FUNCTION_BLOCK FB_EtherCATDiag
VAR_INPUT
	sIPCNetID					: T_AmsNetId; 	// AmsNetId of the IPC 
	sMasterNetID				: T_AmsNetId; 	// AmsNetId of the EtherCAT master device 
	nMasterDevID				: UINT;			// Device ID of EtherCAT master
	nSlaveCount 				: UINT;			// current slave count
	nSlaveCountCfg 				: UINT;			// configured slave count
	nMasterDevState				: WORD;			// device state of EtherCAT Master
	bAllFrameWcStatesOK			: BOOL;			// all FrameWcState OK?
	tTimeout					: TIME := T#5S; // ads timeout
END_VAR
VAR_OUTPUT
	bEtherCATOK					: BOOL;			// no problem on EtherCAT
	bFrameWcStateError			: BOOL;			// error in at least one frame
	bSlaveCountError			: BOOL;			// EtherCAT slave count mismatch (# of cfg slaves <> # of found slaves)
	bMasterDevStateError		: BOOL;			// error in master device state
	stMasterDevState			: ST_EcMasterDevState; // splitted master device state
	bBusy						: BOOL;			// FB busy
	bError						: BOOL;			// FB with error
	iErrorID					: UDINT;		// FB error ID
END_VAR
VAR_IN_OUT
	arrDiagSlaveInfo 			: ARRAY [0..3] OF ST_SlaveStateInfo;		// read in info from configured slaves
	arrDiagSlaveInfoScanned		: ARRAY [0..3] OF ST_SlaveStateInfoScanned;	// read in info from scanned slaves
END_VAR
VAR
	iState						: INT;
	nMasterDevStatePrev			: WORD;
	bSlaveCountErrorPrev		: BOOL;
	bAllFrameWcStatesOKPrev		: BOOL;
	bDiagReq					: BOOL := TRUE;
	I							: UDINT;

	(* -- Get Slave Addresses *)
	fbGetSlaveAddresses 		: FB_EcGetAllSlaveAddr;
	arrSlaveAddresses 			: ARRAY[0..iSLAVEADDR_ARR_SIZE] OF UINT;
	iNumOfSlavesRead			: UINT;

	(* -- Get Slave States *)
	fbGetAllSlaveStates			: FB_EcGetAllSlaveStates;
	arrSlaveStates 				: ARRAY[0..iSLAVEADDR_ARR_SIZE] OF ST_EcSlaveState;

	(* -- Get Topology Data *)
	iTopologyData				: UDINT;
	fbGetTopologyData			: ADSREAD;
	arrTopologyData				: ARRAY[0..iSLAVEADDR_ARR_SIZE] OF ST_TopologyData;

	(* -- Check Topology *)
	iDiagIndex					: ARRAY [0..3] OF UINT;
	iDiagPort					: ARRAY [0..3] OF UINT;
	iIdx						: DINT;

	(* -- Scan Slaves *)
	fbEcGetScannedSlaves		: FB_EcGetScannedSlaves;
	arrScannedSlaveInfo			: ARRAY [0..iSLAVEADDR_ARR_SIZE] OF ST_EcSlaveScannedData;
	nScannedSlaves				: UINT;

	(* -- Get Slave Identities *)
	fbGetSlaveIdentity			: FB_EcGetSlaveIdentity;
	stIdentity 					: ST_EcSlaveIdentity;

	(* -- Get Slave Names *)
	fbGetSlaveName 				: IOF_GetBoxNameByAddr;
	strName						: STRING;

	arrSlaveInfo 				: ARRAY [0..iSLAVEADDR_ARR_SIZE] OF ST_SlaveStateInfo;
	arrSlaveInfoScanned			: ARRAY [0..iSLAVEADDR_ARR_SIZE] OF ST_SlaveStateInfoScanned;
END_VAR

(* cyclic diag *)
bFrameWcStateError := NOT bAllFrameWcStatesOK;

bSlaveCountError := (nSlaveCount <> nSlaveCountCfg) OR (nSlaveCount = 0);
IF (bSlaveCountError AND NOT bSlaveCountErrorPrev) OR (NOT bSlaveCountError AND bSlaveCountErrorPrev) THEN
	bSlaveCountErrorPrev := bSlaveCountError;
	bDiagReq := TRUE; // slave count error change detected --> diag required
END_IF

IF (bAllFrameWcStatesOK AND NOT bAllFrameWcStatesOKPrev) OR (NOT bAllFrameWcStatesOK AND bAllFrameWcStatesOKPrev) THEN
	bAllFrameWcStatesOKPrev := bAllFrameWcStatesOK;
	bDiagReq := TRUE; // frame error change detected --> diag required
END_IF

IF (nMasterDevState <> nMasterDevStatePrev) THEN
	M_CheckMasterDevState();
	bDiagReq := TRUE; // devstate change detected --> diag required
END_IF

(* acyclic diag *)
CASE iState OF
0: (* IDLE *)
	IF bDiagReq THEN				// diag requested
		bDiagReq := FALSE;

		IF sMasterNetID <> '' AND sMasterNetID <> '0.0.0.0.0.0' THEN
			iState := iState + 1;	// execute diag
			bBusy := TRUE;
		ELSE
			bError := TRUE;
			iErrorID := 7;
		END_IF

		bEtherCATOK := FALSE;
	ELSE
		// check for changes in idle
		IF (bSlaveCountError OR bMasterDevStateError OR NOT bAllFrameWcStatesOK) AND NOT (arrSlaveInfo[iDiagIndex[0]].bDiagData) THEN
			bEtherCATOK := FALSE;
			bDiagReq := TRUE;//new error --> diag requested
		ELSIF (bSlaveCountError AND NOT bSlaveCountErrorPrev) OR (NOT bSlaveCountError AND bSlaveCountErrorPrev) THEN
			bSlaveCountErrorPrev := bSlaveCountError;
			bEtherCATOK := FALSE;
			bDiagReq := TRUE;// slave count error change detected --> diag required
		ELSIF (nMasterDevState <> nMasterDevStatePrev) THEN
			bEtherCATOK := FALSE;
			bDiagReq := TRUE;// devstate change detected --> diag required
		ELSIF (bAllFrameWcStatesOK AND NOT bAllFrameWcStatesOKPrev) OR (NOT bAllFrameWcStatesOK AND bAllFrameWcStatesOKPrev) THEN
			bAllFrameWcStatesOKPrev := bAllFrameWcStatesOK;
			bEtherCATOK := FALSE;
			bDiagReq := TRUE;// frame error change detected --> diag required
		ELSIF (bSlaveCountError OR bMasterDevStateError OR NOT bAllFrameWcStatesOK OR arrSlaveInfo[iDiagIndex[0]].bDiagData) THEN
			bEtherCATOK := FALSE;
		ELSE
			bEtherCATOK := TRUE;
		END_IF
	END_IF

1: (* get adresses *)
	M_GetSlaveAdresses();

2: (* get states *)
	M_GetSlaveStates();

3:	(* get topology data length *)
	M_GetTopoDataLen();

4:	(* get topology data *)
	M_GetTopoData();

5:	(* scan slaves *)
	M_ScanSlaves();

6:	(* get identity *)
	M_GetSlaveIdentity();

7:	(* get name *)
	M_GetSlaveName();

8:	(* get scanned name *)
	M_GetScannedSlaveName();

10:	(* DONE *)
	bBusy := FALSE;
	iState := 0;


END_CASE

ACTION M_GetSlaveAdresses:
fbGetSlaveAddresses(
	sNetId		:= sMasterNetID,
	pAddrBuf	:= ADR(arrSlaveAddresses),
	cbBufLen	:= SIZEOF(arrSlaveAddresses),
	bExecute	:= TRUE,
	tTimeout	:= tTimeout,
	nSlaves		=> iNumOfSlavesRead
);

IF NOT fbGetSlaveAddresses.bBusy THEN
	fbGetSlaveAddresses(bExecute:= FALSE);
	IF NOT fbGetSlaveAddresses.bError THEN
		FOR I := 0 TO MIN(iNumOfSlavesRead, iSLAVEADDR_ARR_SIZE) DO
			arrSlaveInfo[I].nECAddr := arrSlaveAddresses[I];
		END_FOR
	END_IF
	iState := iState + 1;
END_IF
END_ACTION

ACTION M_GetSlaveName:
fbGetSlaveName(
	NETID		:= sIPCNetId,
	DEVICEID	:= nMasterDevID,
	BOXADDR		:= arrSlaveInfo[iDiagIndex[iIdx]].nECAddr,
	START		:= TRUE,
	TMOUT		:= tTimeout,
	BOXNAME		=> strName
);

IF NOT fbGetSlaveName.BUSY THEN
	fbGetSlaveName(START:= FALSE);

	IF NOT fbGetSlaveName.ERR THEN
		IF iDiagPort[iIdx] <> 0 THEN
			arrSlaveInfo[iDiagIndex[iIdx]].sName 	:= strName;
		END_IF
	END_IF

	iState := iState + 1;
END_IF
END_ACTION

ACTION M_GetSlaveIdentity:
fbGetSlaveIdentity(
	sNetId		:= sMasterNetID,
	nSlaveAddr	:= arrSlaveInfo[iDiagIndex[iIdx]].nECAddr,
	bExecute	:= TRUE,
	tTimeout	:= tTimeout,
	identity	=> stIdentity
);

IF NOT fbGetSlaveIdentity.bBusy THEN
	fbGetSlaveIdentity(bExecute:= FALSE);

	IF NOT fbGetSlaveIdentity.bError THEN
		IF iDiagPort[iIdx] <> 0 THEN
			arrSlaveInfo[iDiagIndex[iIdx]].nIndex	:= iDiagIndex[iIdx] + 1;
			arrSlaveInfo[iDiagIndex[iIdx]].sType 	:= F_ConvProductCodeToString(stSlaveIdentity := stIdentity);
		END_IF
	END_IF
	iState := iState + 1;
END_IF
END_ACTION

ACTION M_ScanSlaves:
fbEcGetScannedSlaves(
	bExecute				:= TRUE,
	sNetId					:= sMasterNetID,
	pArrEcScannedSlaveInfo	:= ADR(arrScannedSlaveInfo),
	cbBufLen				:= SIZEOF(arrScannedSlaveInfo),
	tTimeout				:= tTimeout
);

IF NOT fbEcGetScannedSlaves.bBusy THEN
	fbEcGetScannedSlaves(bExecute := FALSE);
	iState := iState + 1;

	IF fbEcGetScannedSlaves.bError THEN
		nScannedSlaves := 0;
	ELSE
		nScannedSlaves := fbEcGetScannedSlaves.nSlaves;
	END_IF
END_IF
END_ACTION

ACTION M_GetScannedSlaveName:
fbGetSlaveName(
	NETID		:= sIPCNetId,
	DEVICEID	:= nMasterDevID,
	BOXADDR		:= arrScannedSlaveInfo[iDiagIndex[iIdx]].nAddr,
	START		:= TRUE,
	TMOUT		:= tTimeout,
	BOXNAME		=> strName
);

IF NOT fbGetSlaveName.BUSY THEN
	fbGetSlaveName(START:= FALSE);

	(* add scanned info *)
	arrSlaveInfoScanned[iDiagIndex[iIdx]].nIndex 	:= iDiagIndex[iIdx] + 1;
	IF arrScannedSlaveInfo[iDiagIndex[iIdx]].nAddr <> 0 THEN
		IF NOT fbGetSlaveName.ERR THEN
			arrSlaveInfoScanned[iDiagIndex[iIdx]].sName := strName;
		END_IF
	ELSE
		arrSlaveInfoScanned[iDiagIndex[iIdx]].sType		:= '';
	END_IF

	IF (iDiagIndex[iIdx] < nScannedSlaves) THEN
		arrSlaveInfoScanned[iDiagIndex[iIdx]].sType		:= F_ConvProductCodeToString(arrScannedSlaveInfo[iDiagIndex[iIdx]].stSlaveIdentity);
	ELSE
		arrSlaveInfoScanned[iDiagIndex[iIdx]].sType		:= '';
	END_IF

	arrSlaveInfoScanned[iDiagIndex[iIdx]].nECAddr	:= arrScannedSlaveInfo[iDiagIndex[iIdx]].nAddr;

	IF arrSlaveInfoScanned[iDiagIndex[iIdx]].sName <> arrSlaveInfo[iDiagIndex[iIdx]].sName THEN
		arrSlaveInfoScanned[iDiagIndex[iIdx]].bDifferentName := TRUE;
	ELSE
		arrSlaveInfoScanned[iDiagIndex[iIdx]].bDifferentName := FALSE;
	END_IF

	IF arrSlaveInfoScanned[iDiagIndex[iIdx]].nECAddr <> arrSlaveInfo[iDiagIndex[iIdx]].nECAddr THEN
		arrSlaveInfoScanned[iDiagIndex[iIdx]].bDifferentAddr := TRUE;
	ELSE
		arrSlaveInfoScanned[iDiagIndex[iIdx]].bDifferentAddr := FALSE;
	END_IF

	IF arrSlaveInfoScanned[iDiagIndex[iIdx]].sType <> arrSlaveInfo[iDiagIndex[iIdx]].sType THEN
		arrSlaveInfoScanned[iDiagIndex[iIdx]].bDifferentType := TRUE;
	ELSE
		arrSlaveInfoScanned[iDiagIndex[iIdx]].bDifferentType := FALSE;
	END_IF

	IF iIdx < 3 THEN
		iIdx := iIdx + 1;
		iState := iState - 2;
	ELSE
		iIdx := 0;
		iState := 10;

		FOR I := 0 TO 3 DO
			IF iDiagPort[I] <> 0 THEN
				arrDiagSlaveInfo[I] := arrSlaveInfo[iDiagIndex[I]];
				arrDiagSlaveInfoScanned[I] := arrSlaveInfoScanned[iDiagIndex[I]];
			ELSE
				MEMSET(ADR(arrDiagSlaveInfo[I]), 0, SIZEOF(arrDiagSlaveInfo[I]));
				MEMSET(ADR(arrDiagSlaveInfoScanned[I]), 0, SIZEOF(arrDiagSlaveInfoScanned[I]));
			END_IF
		END_FOR
	END_IF
END_IF
END_ACTION

ACTION M_CheckMasterDevState:
(* check master errors based on devstate *)
bMasterDevStateError 				:= nMasterDevState <> 0;
stMasterDevState.bLinkError 		:= ((nMasterDevState AND 16#000F) = 1) OR ((nMasterDevState AND 16#000F) = 4);
stMasterDevState.bResetRequired 	:= ((nMasterDevState AND 16#000F) = 2) OR ((nMasterDevState AND 16#FFF0) = 16#10);
stMasterDevState.bMissFrmRedMode 	:= (nMasterDevState AND 16#000F) = 8;
stMasterDevState.bWatchdogTriggerd 	:= (nMasterDevState AND 16#20) = 16#20;
stMasterDevState.bDriverNotFound 	:= (nMasterDevState AND 16#40) = 16#40;
stMasterDevState.bResetActive 		:= (nMasterDevState AND 16#80) = 16#80;
stMasterDevState.bAtLeastOneNotInOp := ((nMasterDevState AND 16#100) = 16#100) OR ((nMasterDevState AND 16#200) = 16#200) OR
										((nMasterDevState AND 16#400) = 16#400) OR ((nMasterDevState AND 16#800) = 16#800);
stMasterDevState.bDcNotInSync 		:= (nMasterDevState AND 16#1000) = 16#1000;
nMasterDevStatePrev 				:= nMasterDevState;
END_ACTION

ACTION M_GetTopoData:
fbGetTopologyData(
	NETID	:= sMasterNetID,
	PORT	:= 16#FFFF,
	IDXGRP	:= 16#22,
	IDXOFFS	:= 0,
	LEN		:= iTopologyData*SIZEOF(arrTopologyData[0]),
	DESTADDR:= ADR(arrTopologyData),
	READ	:= TRUE,
	TMOUT	:= tTimeout,
);

IF NOT fbGetTopologyData.BUSY THEN
	fbGetTopologyData(READ := FALSE);

	IF NOT fbGetTopologyData.ERR THEN
		iDiagPort[0] := arrTopologyData[iDiagIndex[0]].iOwnPhysicalAddr;
		iDiagPort[1] := arrTopologyData[iDiagIndex[0]].stPhysicalAddr.portB;
		iDiagPort[2] := arrTopologyData[iDiagIndex[0]].stPhysicalAddr.portC;
		iDiagPort[3] := arrTopologyData[iDiagIndex[0]].stPhysicalAddr.portD;

		(* clear diag index  *)
		iDiagIndex[1] := 0;
		iDiagIndex[2] := 0;
		iDiagIndex[3] := 0;

		(* find slaves on PortB of first slave with diag *)
		IF iDiagPort[1] <> 0 THEN
			FOR I := 0 TO MIN(iTopologyData-1,iSLAVEADDR_ARR_SIZE) DO
				IF arrTopologyData[I].iOwnPhysicalAddr = iDiagPort[1] THEN
					iDiagIndex[1] := UDINT_TO_UINT(I);
					EXIT;
				END_IF
			END_FOR
		END_IF

		(* find slaves on PortC of first slave with diag *)
		IF iDiagPort[2] <> 0 THEN
			FOR I := 0 TO MIN(iTopologyData-1,iSLAVEADDR_ARR_SIZE) DO
				IF arrTopologyData[I].iOwnPhysicalAddr = iDiagPort[2] THEN
					iDiagIndex[2] := UDINT_TO_UINT(I);
					EXIT;
				END_IF
			END_FOR
		END_IF

		(* find slaves on PortD of first slave with diag *)
		IF iDiagPort[3] <> 0 THEN
			FOR I := 0 TO MIN(iTopologyData-1,iSLAVEADDR_ARR_SIZE) DO
				IF arrTopologyData[I].iOwnPhysicalAddr = iDiagPort[3] THEN
					iDiagIndex[3] := UDINT_TO_UINT(I);
					EXIT;
				END_IF
			END_FOR
		END_IF
	END_IF

	iIdx := 0;
	iState := iState + 1;
END_IF
END_ACTION

ACTION M_GetSlaveStates:
fbGetAllSlaveStates(
	sNetId		:= sMasterNetID,
	pStateBuf	:= ADR(arrSlaveStates),
	cbBufLen	:= SIZEOF(arrSlaveStates),
	bExecute	:= TRUE,
	tTimeout	:= tTimeout,
	nSlaves		=> iNumOfSlavesRead
);

IF NOT fbGetAllSlaveStates.bBusy THEN
	fbGetAllSlaveStates(bExecute:= FALSE);

	IF NOT fbGetAllSlaveStates.bError THEN
		IF iNumOfSlavesRead = nSlaveCountCfg THEN
			FOR I := 0 TO 3 DO
				iDiagIndex[I] := 0;
			END_FOR

			(* split slave state and link state *)
			FOR I := 0 TO MIN(iNumOfSlavesRead, iSLAVEADDR_ARR_SIZE) DO
				(* slave state*)
				arrSlaveInfo[I].stState.eEcState 		:= arrSlaveStates[I].deviceState AND 16#0F;
				arrSlaveInfo[I].stState.bError 			:= arrSlaveStates[I].deviceState.4;
				arrSlaveInfo[I].stState.bInvalidVPRS 	:= arrSlaveStates[I].deviceState.5;
				(* link state *)
				arrSlaveInfo[I].stState.bNoCommToSlave 	:= arrSlaveStates[I].linkState.0;
				arrSlaveInfo[I].stState.bLinkError 		:= arrSlaveStates[I].linkState.1;
				arrSlaveInfo[I].stState.bMissingLink 	:= arrSlaveStates[I].linkState.2;
				arrSlaveInfo[I].stState.bUnexpectedLink := arrSlaveStates[I].linkState.3;
				arrSlaveInfo[I].stState.bPortA 			:= arrSlaveStates[I].linkState.4;
				arrSlaveInfo[I].stState.bPortB 			:= arrSlaveStates[I].linkState.5;
				arrSlaveInfo[I].stState.bPortC 			:= arrSlaveStates[I].linkState.6;
				arrSlaveInfo[I].stState.bPortD 			:= arrSlaveStates[I].linkState.7;
				(* DiagData *)
				arrSlaveInfo[I].bDiagData	:= ((arrSlaveStates[I].deviceState AND 16#F0) <> 0) OR
					(((arrSlaveStates[I].deviceState AND 16#0F) > 0) AND ((arrSlaveStates[I].deviceState AND 16#0F) < 8)) OR
					(arrSlaveStates[I].linkState <> 0);

				IF arrSlaveInfo[I].bDiagData THEN
					IF (I=0) THEN
						iDiagIndex[0] := 0;
					ELSE
						IF (iDiagIndex[0] = 0) AND NOT arrSlaveInfo[0].bDiagData THEN
							iDiagIndex[0] :=  UDINT_TO_UINT(I);
						END_IF
					END_IF
				END_IF
			END_FOR
		END_IF
	END_IF

	IF arrSlaveInfo[iDiagIndex[0]].bDiagData THEN
		iState := iState + 1;
	ELSE
		FOR I := 0 TO 3 DO
			MEMSET(ADR(arrDiagSlaveInfo[I]), 0, SIZEOF(arrDiagSlaveInfo[I]));
			MEMSET(ADR(arrDiagSlaveInfoScanned[I]), 0, SIZEOF(arrDiagSlaveInfoScanned[I]));
		END_FOR
		iState := 10;
	END_IF
END_IF
END_ACTION

ACTION M_GetTopoDataLen:
fbGetTopologyData(
	NETID	:= sMasterNetID,
	PORT	:= 16#FFFF,
	IDXGRP	:= EC_ADS_IGRP_MASTER_COUNT_SLAVE,
	IDXOFFS	:= EC_ADS_IOFFS_MASTER_COUNT_SLAVE,
	LEN		:= SIZEOF(iTopologyData),
	DESTADDR:= ADR(iTopologyData),
	READ	:= TRUE,
	TMOUT	:= tTimeout,
);

IF NOT fbGetTopologyData.BUSY THEN
	fbGetTopologyData(READ := FALSE);

	iState := iState + 1;
END_IF
END_ACTION

END_FUNCTION_BLOCK
